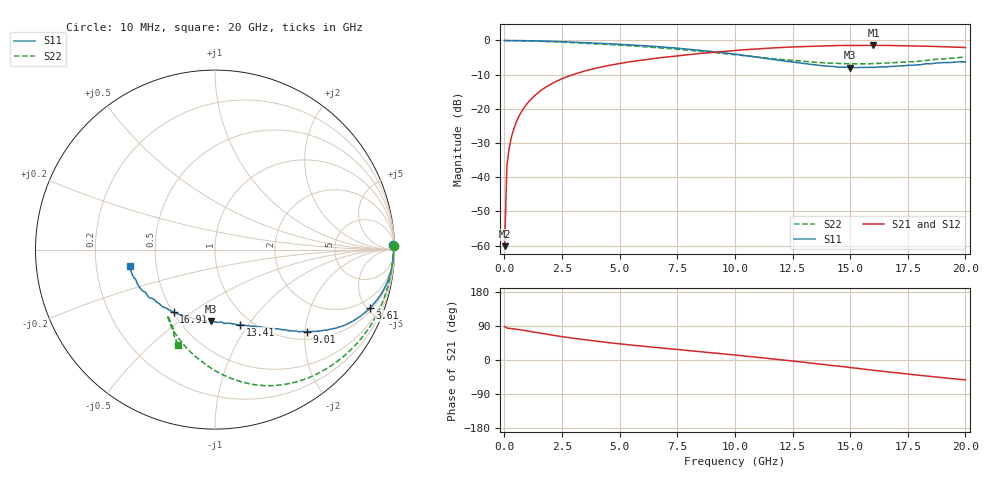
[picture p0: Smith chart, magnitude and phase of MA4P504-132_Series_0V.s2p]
! AWR Design Environment (9226) Thu Aug 19 02:45:16 2021
! Document = '0V'
! nPorts: 2, nXvals: 201
# GHz S DB R 50
!Freq DBS11 AngS11 DBS21 AngS21 DBS12 AngS12 DBS22 AngS22
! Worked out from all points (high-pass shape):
!   201 points, 10 MHz to 20 GHz, reference 50 ohm
!   highest |S21| = -1.45 dB at 16.01 GHz (marker M1); lowest = -60.2 dB at 10 MHz (marker M2)
!   |S21| within 3 dB of the highest: 7.569 GHz to end of sweep
!   lowest |S11| = -8.0 dB at 15.01 GHz (marker M3), VSWR 2.33, Z = 34.9 - j33.1 ohm
!   |S11| at or under -10 dB: nowhere
!   |S22| runs from -6.9 to 0.0 dB; largest |S21 - S12| = 0.029
!   S11 on the Smith chart (normalised r, x): 10 MHz: 20, +82; 3.61 GHz: 1.20, -5.22; 9.01 GHz: 1.18, -2.05; 13.41 GHz: 0.88, -0.91; 16.91 GHz: 0.50, -0.43; 20 GHz: 0.35, -0.08
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0.01  -0.05 1.3  -60.20 88.1  -56.78 72.1  -0.03 1.3
0.11  -0.05 -0.8  -36.68 84.4  -36.86 84.0  -0.07 -1.8
0.21  -0.04 -1.5  -31.41 83.6  -31.43 83.7  -0.08 -3.3
0.31  -0.05 -2.2  -28.20 82.9  -28.20 83.0  -0.09 -4.9
0.51  -0.06 -3.5  -24.02 81.4  -24.04 81.4  -0.11 -8.0
0.91  -0.09 -6.0  -19.18 77.4  -19.19 77.5  -0.15 -14.1
1.51  -0.18 -9.8  -15.05 71.2  -15.07 71.5  -0.26 -22.9
2.31  -0.34 -14.3  -11.80 63.4  -11.81 63.8  -0.47 -33.7
3.41  -0.64 -19.8  -9.11 53.9  -9.11 54.5  -0.82 -46.5
3.61  -0.70 -20.7  -8.74 52.4  -8.74 53.0  -0.89 -48.6
5.01  -1.17 -26.4  -6.76 42.7  -6.76 43.3  -1.40 -61.4
6.71  -1.86 -32.7  -5.12 32.4  -5.09 33.3  -2.16 -74.4
9.01  -3.27 -41.8  -3.53 19.3  -3.47 20.3  -3.50 -90.9
10.01  -4.04 -46.2  -2.95 13.1  -2.89 14.3  -4.19 -98.5
11.71  -5.64 -56.3  -2.19 2.4  -2.13 3.5  -5.38 -111.6
13.41  -7.10 -71.7  -1.71 -8.8  -1.66 -7.8  -6.36 -121.5
15.01  -7.97 -93.3  -1.48 -20.0  -1.48 -18.8  -6.84 -125.2
16.01  -7.90 -108.5  -1.45 -27.0  -1.46 -25.3  -6.80 -124.4
16.71  -7.64 -119.8  -1.49 -31.8  -1.50 -30.0  -6.60 -122.5
16.91  -7.58 -123.3  -1.51 -33.0  -1.51 -31.4  -6.52 -121.8
18.91  -6.55 -154.2  -1.80 -46.0  -1.81 -44.6  -5.48 -115.2
20  -6.32 -169.2  -2.09 -52.6  -2.13 -51.3  -4.86 -111.3
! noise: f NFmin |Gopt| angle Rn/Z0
0.01  0  1  0  2e-20
2.21  0  1  0  2e-20
4.41  0  1  0  2e-20
6.61  0  1  0  2e-20
8.81  0  1  0  2e-20
11.11  0  1  0  2e-20
13.31  0  1  0  2e-20
15.51  0  1  0  2e-20
17.71  0  1  0  2e-20
20  0  1  0  2e-20
